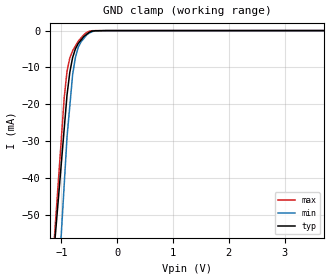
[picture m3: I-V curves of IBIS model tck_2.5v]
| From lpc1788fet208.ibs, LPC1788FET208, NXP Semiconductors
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[Model] tck_2.5v
Model_type Input
Vinl = 750.000mV
Vinh = 1.75000V
C_comp 983.000fF 934.000fF 1030.000fF
| variable typ   min   max
[Voltage Range] 2.50000V 2.40000V 2.60000V
[POWER Clamp Reference] 2.50000V 2.40000V 2.60000V
[GND Clamp Reference] 0.00000V 0.00000V 0.00000V
[Temperature Range]   25   85   -40
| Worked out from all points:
|   GND clamp passes 1 mA (typ) near -0.55 V on its own axis
[GND Clamp]
-2.5V     -307.9mA   -438.9mA   -352.4mA
-950mV    -26.53mA   -41.68mA   -18.15mA
-900mV    -17.46mA   -28.86mA   -11mA
-850mV    -11.31mA   -20.43mA   -7.42mA
-800mV    -7.334mA   -11.99mA   -5.484mA
-750mV    -4.977mA   -7.285mA   -4.187mA
-700mV    -3.511mA   -4.557mA   -2.89mA
-650mV    -2.574mA   -3.076mA   -2.012mA
-550mV    -1.038mA   -1.207mA   -522.6uA
-400mV    -38.64uA   -91.5uA    -27.74uA
-200mV    -2.076uA   -5.905uA   -1.88uA
5V        2.337uA    4.528uA    2.676uA
[POWER Clamp]
-2.5V     0A         0A         0A
5V        0A         0A         0A
